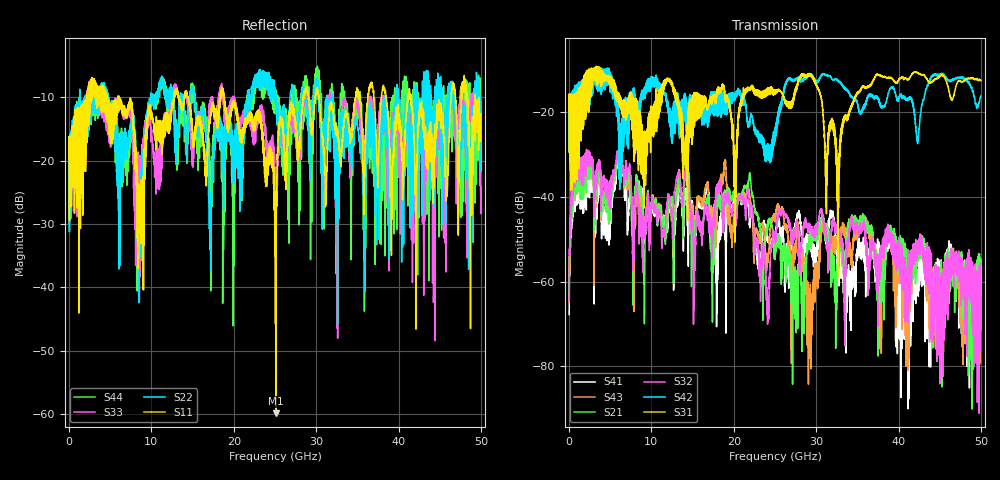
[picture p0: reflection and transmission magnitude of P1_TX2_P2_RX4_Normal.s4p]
!Keysight Technologies,N5225B,MY57041031,A.13.20.10
!Date: Friday, May 31, 2019 11:33:24
!Correction: S11(Full 4 Port(1,2,3,4))
!S12(Full 4 Port(1,2,3,4))
!S13(Full 4 Port(1,2,3,4))
!S14(Full 4 Port(1,2,3,4))
!S21(Full 4 Port(1,2,3,4))
!S22(Full 4 Port(1,2,3,4))
!S23(Full 4 Port(1,2,3,4))
!S24(Full 4 Port(1,2,3,4))
!S31(Full 4 Port(1,2,3,4))
!S32(Full 4 Port(1,2,3,4))
!S33(Full 4 Port(1,2,3,4))
!S34(Full 4 Port(1,2,3,4))
!S41(Full 4 Port(1,2,3,4))
!S42(Full 4 Port(1,2,3,4))
!S43(Full 4 Port(1,2,3,4))
!S44(Full 4 Port(1,2,3,4))
!S4P File: Measurements: <S11,S12,S13,S14>,
!<S21,S22,S23,S24>,
!<S31,S32,S33,S34>,
!<S41,S42,S43,S44>:
# Hz S  dB  R 50.0
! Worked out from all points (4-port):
!   5000 points, 10 MHz to 50 GHz, reference 50 ohm
!   strongest paths, dB at 10 MHz, 12.51 GHz, 25.01 GHz, 37.51 GHz, 50 GHz:
!     S31: -19.5, -13.0, -15.5, -11.1, -12.5
!     S42: -19.7, -27.4, -23.8, -16.9, -16.2
!     S32: -64.6, -43.8, -49.7, -58.7, -63.3
!     S21: -59.7, -39.9, -54.3, -64.4, -56.6
!     S43: -59.0, -43.9, -44.8, -58.0, -58.9
!     S41: -67.8, -41.3, -50.5, -51.7, -57.4
!   lowest |S11| = -59.9 dB at 25.1 GHz (marker M1), VSWR 1.00, Z = 49.9 + j0.0742 ohm
!   |S11| at or under -10 dB: 6.091 GHz to 12.71 GHz (6.616 GHz wide, 70.4 % of centre); 18.82 GHz to 28.43 GHz (9.605 GHz wide, 40.7 % of centre); 41.58 GHz to 46.38 GHz (4.809 GHz wide, 10.9 % of centre)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
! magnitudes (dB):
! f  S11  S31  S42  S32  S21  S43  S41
! 10 MHz  -19.8  -19.5  -19.7  -64.6  -59.7  -59.0  -67.8
! 6 GHz  -11.4  -16.5  -24.5  -30.3  -30.5  -31.2  -31.7
! 25.1 GHz  -59.9  -15.1  -24.7  -48.9  -50.5  -43.8  -47.8
! 29.17 GHz  -11.3  -11.1  -11.4  -47.1  -50.1  -70.6  -49.5
! 32.64 GHz  -15.8  -37.1  -12.5  -49.0  -55.3  -51.8  -55.2
! 35.73 GHz  -20.5  -13.9  -19.2  -46.1  -45.4  -45.0  -52.9
! 50 GHz  -12.6  -12.5  -16.2  -63.3  -56.6  -58.9  -57.4
